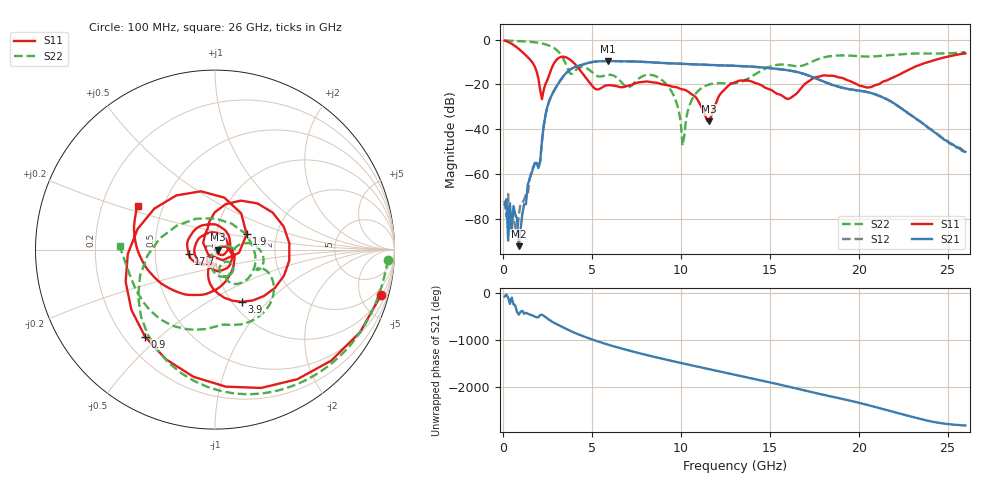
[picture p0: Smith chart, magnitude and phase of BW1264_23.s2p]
!Keysight Technologies,N5245B,MY57181159,A.13.60.06
!Date: Friday, December 18, 2020 23:53:07
!Correction: S11(Full 2 Port(1,2))
!S21(Full 2 Port(1,2))
!S12(Full 2 Port(1,2))
!S22(Full 2 Port(1,2))
!S2P File: Measurements: S11, S21, S12, S22:
# Hz S  dB  R 50
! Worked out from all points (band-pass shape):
!   260 points, 100 MHz to 26 GHz, reference 50 ohm
!   highest |S21| = -9.54 dB at 5.9 GHz (marker M1); lowest = -92.4 dB at 900 MHz (marker M2)
!   |S21| within 3 dB of the highest: 3.964 GHz to 14.81 GHz (10.84 GHz wide, 116 % of centre)
!   lowest |S11| = -36.5 dB at 11.6 GHz (marker M3), VSWR 1.03, Z = 51.5 + j0.0054 ohm
!   |S11| at or under -10 dB: 1.643 GHz to 2.92 GHz (1.277 GHz wide, 56 % of centre); 3.94 GHz to 23.9 GHz (19.96 GHz wide, 143 % of centre)
!   |S22| runs from -47.3 to -0.3 dB; largest |S21 - S12| = 0.00061
!   S11 on the Smith chart (normalised r, x): 100 MHz: 1.15, -7.24; 900 MHz: 0.28, -0.45; 1.9 GHz: 1.40, +0.25; 3.9 GHz: 1.11, -0.72; 17.7 GHz: 0.74, -0.04; 26 GHz: 0.36, +0.23
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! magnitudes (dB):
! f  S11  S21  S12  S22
! 100 MHz  -0.4  -73.7  -72.1  -0.3
! 200 MHz  -0.6  -71.4  -79.2  -0.4
! 300 MHz  -1.0  -89.9  -69.1  -0.4
! 400 MHz  -1.4  -73.2  -85.2  -0.4
! 900 MHz  -4.1  -92.4  -78.2  -0.6
! 1.9 GHz  -14.2  -55.1  -55.1  -1.2
! 2.2 GHz  -26.6  -45.2  -45.3  -1.6
! 2.7 GHz  -13.7  -25.7  -25.7  -2.9
! 3.9 GHz  -9.7  -12.8  -12.8  -15.3
! 4.5 GHz  -15.3  -11.1  -11.1  -12.2
! 5.9 GHz  -20.3  -9.5  -9.5  -15.7
! 8.8 GHz  -19.6  -10.3  -10.3  -17.2
! 9.7 GHz  -21.1  -10.7  -10.7  -26.8
! 10.1 GHz  -22.2  -10.8  -10.8  -47.3
! 10.6 GHz  -24.3  -11.0  -11.0  -27.3
! 11.6 GHz  -36.5  -11.3  -11.3  -20.0
! 13.1 GHz  -18.9  -11.7  -11.7  -19.3
! 16 GHz  -26.5  -13.6  -13.6  -11.3
! 17.4 GHz  -17.4  -16.7  -16.7  -9.7
! 17.7 GHz  -16.6  -17.7  -17.7  -8.7
! 21.7 GHz  -17.7  -27.1  -27.1  -6.9
! 26 GHz  -6.1  -50.2  -50.0  -5.5
